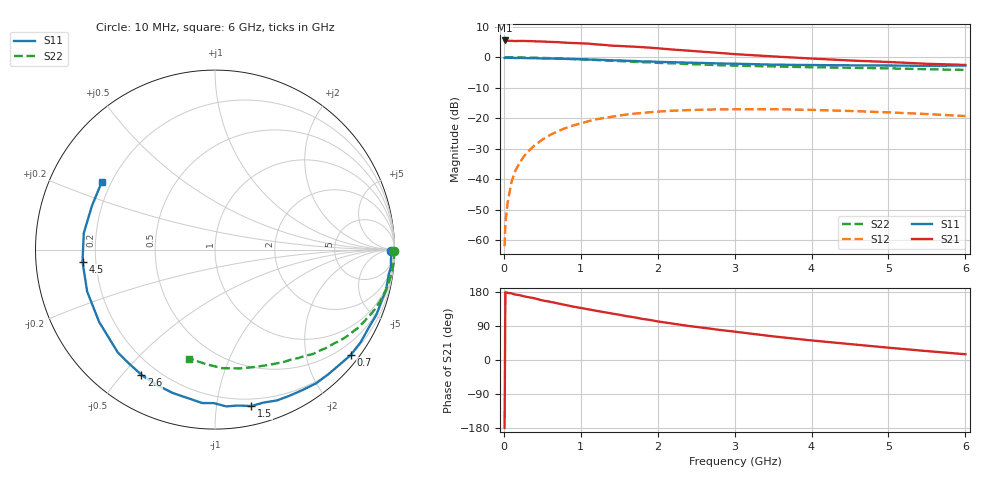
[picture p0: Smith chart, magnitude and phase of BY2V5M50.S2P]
! SIEMENS Small Signal Semiconductors
! BFY420
! Si NPN RF SIEGET Grounded Emitter Transistor in MICRO-X
! VCE = 2.5 V  IC = 0.5 mA
! Common Emitter S-Parameters:  October  1996
# GHz  S  MA  R  50
!  f  S11  S21  S12  S22
! GHz  MAG  ANG  MAG  ANG  MAG  ANG  MAG  ANG
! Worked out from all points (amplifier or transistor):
!   36 points, 10 MHz to 6 GHz, reference 50 ohm
!   highest |S21| = 5.6 dB at 10 MHz (marker M1)
!   |S21| within 3 dB of that: start of sweep to 2.204 GHz
!   unconditionally stable (mu >= 1): 4.729 GHz to end of sweep
!   at 250 MHz: K = 0.02, MSG = 19.1 dB, |S12| = -32.9 dB
!   at 1.4 GHz: K = 0.18, MSG = 11.7 dB, |S12| = -19.5 dB
!   at 6 GHz: K = 1.42, MAG = 4.5 dB, |S12| = -19.3 dB
!   S11 on the Smith chart (normalised r, x): 10 MHz: 75, -37; 700 MHz: 0.21, -2.91; 1.5 GHz: 0.14, -1.25; 2.6 GHz: 0.14, -0.56; 4.5 GHz: 0.15, -0.04; 6 GHz: 0.16, +0.27
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0.01  0.9787 -0.6  1.897 -179.2  0.0008 85.6  0.9999 -0.3
0.02  0.9833 -1.4  1.894 178.8  0.0019 96.5  0.9974 -0.4
0.05  0.9817 -2.9  1.868 177.2  0.0042 90.8  0.9986 -1.3
0.1  0.9852 -5.6  1.873 175.9  0.0091 87.2  0.9982 -2.6
0.15  0.9777 -8.1  1.853 172.7  0.0139 84.1  0.9967 -3.9
0.3  0.9724 -16.1  1.854 166.4  0.0275 80.1  0.9926 -7.6
0.4  0.9701 -21.8  1.839 162.8  0.036 76.3  0.9862 -10.2
0.5  0.9605 -27.0  1.82 157.2  0.0448 73.0  0.9806 -12.7
0.7  0.9574 -37.8  1.779 149.5  0.0612 67.0  0.9626 -17.6
0.9  0.9386 -47.9  1.722 140.9  0.0763 59.4  0.9415 -22.2
1.1  0.9219 -58.1  1.682 133.7  0.0897 53.6  0.9183 -26.6
1.5  0.8947 -76.9  1.542 119.4  0.111 42.0  0.8711 -34.6
1.8  0.8553 -90.5  1.472 108.5  0.1227 34.4  0.8353 -39.9
2.2  0.8328 -106.5  1.344 95.9  0.1337 25.0  0.7984 -46.7
2.6  0.8094 -120.4  1.235 84.9  0.1386 17.4  0.7616 -52.5
3  0.7884 -133.4  1.132 74.8  0.1408 10.5  0.7346 -58.3
3.5  0.761 -148.0  1.038 62.4  0.1415 3.3  0.7099 -64.8
4  0.7497 -161.8  0.958 51.6  0.1377 -2.6  0.6896 -71.6
4.5  0.7412 -174.8  0.89 42.0  0.1321 -7.8  0.6758 -78.6
5  0.7368 172.9  0.841 32.5  0.1253 -11.3  0.6615 -86.6
5.5  0.7277 160.7  0.786 23.5  0.1177 -13.6  0.6399 -94.5
6  0.7353 149.0  0.753 15.2  0.109 -13.8  0.6239 -103.3
